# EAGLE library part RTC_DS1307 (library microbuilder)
DS1307 I2C RTC with 56-Bytes RAM
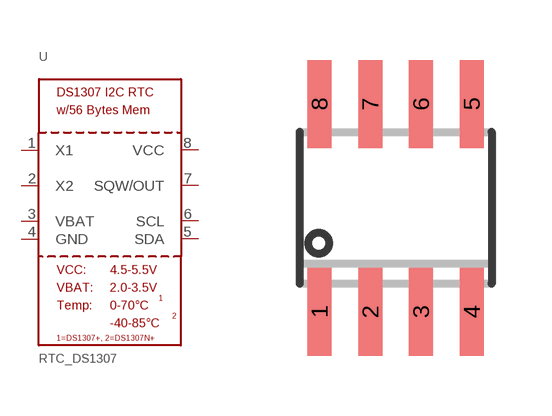
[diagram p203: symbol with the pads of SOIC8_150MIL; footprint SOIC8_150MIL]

Designator prefix U

## RTC_DS1307  [SOIC8_150MIL]
1  X1
2  X2
3  VBAT
4  GND
5  SDA
6  SCL
7  SQW/OUT
8  VCC

## Footprint SOIC8_150MIL (pad centres in mm)
Small Outline IC - 150mil Wide
smd 0.6 x 2.2: 1 -1.905,-2.6; 2 -0.635,-2.6; 3 0.635,-2.6; 4 1.905,-2.6; 5 1.905,2.6; 6 0.635,2.6; 7 -0.635,2.6; 8 -1.905,2.6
